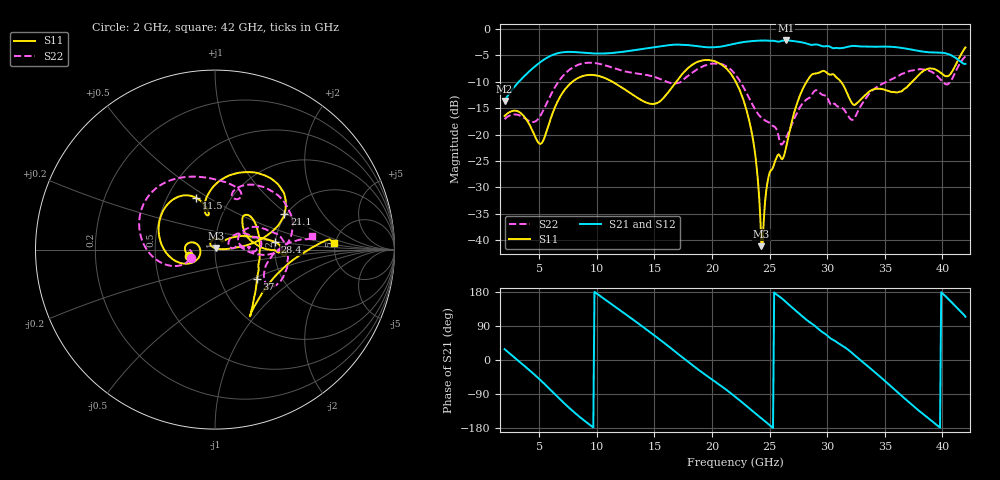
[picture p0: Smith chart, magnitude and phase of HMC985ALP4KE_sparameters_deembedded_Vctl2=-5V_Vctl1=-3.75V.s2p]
!s2p File: Measurements: S11, S21, S12, S22
# GHz S dB R 50.0
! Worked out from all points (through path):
!   401 points, 2 GHz to 42 GHz, reference 50 ohm
!   highest |S21| = -2.24 dB at 26.4 GHz (marker M1); lowest = -13.7 dB at 2 GHz (marker M2)
!   lowest |S11| = -41.1 dB at 24.3 GHz (marker M3), VSWR 1.02, Z = 50.5 + j0.709 ohm
!   |S11| at or under -10 dB: start of sweep to 7.911 GHz; 22.06 GHz to 28.23 GHz (6.174 GHz wide, 24.6 % of centre); 31.18 GHz to 37.39 GHz (6.204 GHz wide, 18.1 % of centre)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
!   |S22| runs from -21.9 to -5.3 dB; largest |S21 - S12| = 0.00094
!   S11 on the Smith chart (normalised r, x): 2 GHz: 0.75, -0.06; 11.5 GHz: 0.69, +0.44; 21.1 GHz: 1.95, +0.95; 28.4 GHz: 2.00, +0.19; 37 GHz: 1.50, -0.53; 42 GHz: 4.85, +0.65
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2  -16.50 -165.7  -13.65 28.6  -13.66 28.6  -17.10 -161.4
3.4  -15.96 169.0  -9.67 -7.4  -9.67 -7.4  -16.49 -178.6
5.1  -21.78 -174.7  -6.34 -52.7  -6.34 -52.7  -16.46 -159.2
6.3  -15.23 -153.0  -4.87 -88.2  -4.87 -88.2  -11.33 -161.0
8.7  -9.03 149.2  -4.54 -154.7  -4.54 -154.7  -6.62 151.7
11.5  -10.22 110.3  -4.58 142.7  -4.58 142.7  -7.47 106.0
13.6  -13.17 100.2  -3.97 96.5  -3.97 96.5  -8.52 77.3
15.4  -13.88 104.4  -3.39 55.7  -3.39 55.7  -9.44 64.1
17.9  -7.50 78.9  -3.12 -4.2  -3.12 -4.2  -8.97 71.1
21.1  -7.25 27.0  -3.27 -75.2  -3.27 -75.2  -6.96 15.7
22  -9.76 16.9  -2.85 -96.5  -2.85 -96.5  -8.58 0.7
23.5  -20.16 4.7  -2.36 -133.8  -2.36 -133.8  -14.28 -4.1
24.3  -41.08 52.6  -2.27 -154.0  -2.26 -153.9  -16.84 6.1
25  -27.25 127.5  -2.29 -171.7  -2.29 -171.7  -17.78 10.0
26.4  -22.82 44.4  -2.24 153.5  -2.24 153.6  -20.75 32.0
28.4  -9.42 7.1  -2.95 101.5  -2.95 101.5  -13.15 18.4
28.7  -8.64 2.0  -3.08 95.4  -3.08 95.4  -12.38 16.7
32.4  -14.40 29.8  -3.28 12.2  -3.28 12.2  -16.79 26.7
35.4  -11.83 17.1  -3.42 -65.7  -3.42 -65.6  -9.80 18.5
37  -10.88 -34.7  -3.84 -108.8  -3.84 -108.7  -8.12 4.4
39.8  -8.26 -55.7  -4.54 -178.6  -4.54 -178.5  -9.50 -33.2
42  -3.56 3.2  -6.66 114.2  -6.66 114.3  -5.26 8.1
